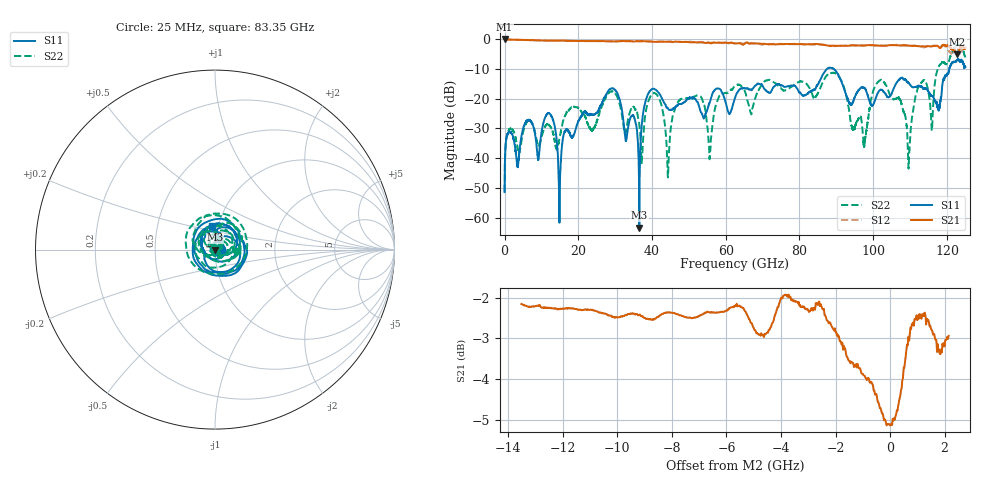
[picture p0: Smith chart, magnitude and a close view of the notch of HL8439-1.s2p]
! 3/1/2024 12:49:34 PM
! H:\PROTOTYPE_DATA\AMOTECH 110G\GROUND WITH BIGGER HOLE.S2P
! CHANNEL.1
! TR.MEASUREMENT
! CORRECTED.DATA
! RF.CORRECTION: FULL.TWO.PORT.CAL.PORT.1.2
! AVERAGING: 1 PointByPoint
! IF.BANDWIDTH: 1KHZ
! SWEEPTYPE:  FREQ.SWEEP(Linear)
! Reference Plane Port Info
! PORT:  PORT1  PORT2
! DISTANCE:  0  m  0  m
! TIME:  0  s  0  s
! PHASE.OFFSET:  0 °  0 °
! LOSS:  0  dB  0  dB
! REF.LOSS:  0  dB  0  dB
! REF.FREQ:  0  Hz  0  Hz
! Power Info
! POWER:  -10  dBm  -10  dBm
! EFF.POWER:  -10  dBm  -10  dBm
! POWER(>54G):  -10  dBm  -10  dBm
! EFF.POWER(>54G):  -10  dBm  -10  dBm
! SOURCE.ATTEN:  0  dB  0  dB
! TEST.ATTEN:  0  dB  0  dB
# GHZ S RI R 50.0
! FREQ.GHZ  S11RE  S11IM  S21RE  S21IM  S12RE  S12IM  S22RE  S22IM
!; PortSelection: Port_12
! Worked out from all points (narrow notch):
!   5000 points, 25 MHz to 125 GHz, reference 50 ohm
!   highest |S21| = -0.01 dB at 25 MHz (marker M1); lowest = -5.1 dB at 122.8 GHz (marker M2)
!   notch at M2: 3.8 dB deep, 2.26 GHz wide at half that depth
!   lowest |S11| = -63.3 dB at 36.55 GHz (marker M3), VSWR 1.00, Z = 50 - j0.0675 ohm
!   |S11| at or under -10 dB: start of sweep to 87.5 GHz; 89.27 GHz to 120.6 GHz (31.37 GHz wide, 29.9 % of centre)
!   |S22| runs from -51.2 to -1.8 dB; largest |S21 - S12| = 0.2
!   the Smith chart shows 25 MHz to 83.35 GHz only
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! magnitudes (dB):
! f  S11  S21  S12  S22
! 25 MHz  -51.4  0.0  0.0  -51.2
! 1.375 GHz  -31.2  -0.2  -0.2  -30.3
! 9.175 GHz  -40.6  -0.4  -0.5  -35.8
! 11.95 GHz  -24.9  -0.5  -0.5  -28.8
! 14.97 GHz  -52.4  -0.5  -0.5  -32.7
! 20.88 GHz  -25.9  -0.6  -0.7  -24.5
! 29.68 GHz  -16.7  -0.8  -0.8  -17.9
! 36.55 GHz  -63.3  -0.7  -0.7  -28.5
! 41.7 GHz  -17.9  -0.9  -0.9  -19.5
! 44.35 GHz  -23.4  -0.9  -0.9  -45.9
! 47.5 GHz  -21.8  -0.9  -0.9  -20.4
! 55.67 GHz  -21.1  -1.4  -1.2  -39.3
! 62.52 GHz  -19.5  -1.5  -1.4  -15.7
! 83.35 GHz  -17.3  -1.8  -1.7  -18.2
! 90.05 GHz  -11.0  -2.3  -2.4  -11.8
! 97.67 GHz  -16.5  -2.2  -2.2  -34.3
! 104.2 GHz  -19.5  -2.1  -2.1  -17.7
! 109.7 GHz  -14.9  -2.2  -2.2  -39.9
! 112.4 GHz  -15.7  -2.4  -2.5  -15.6
! 115.8 GHz  -19.1  -2.4  -2.3  -30.2
! 122.8 GHz  -7.0  -5.1  -3.1  -2.0
! 125 GHz  -9.4  -2.9  -3.2  -6.4
